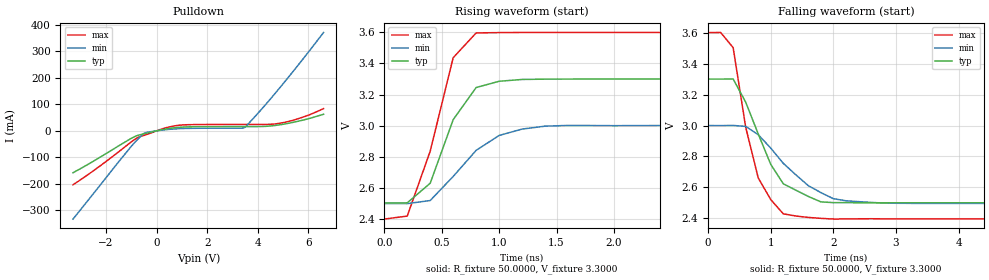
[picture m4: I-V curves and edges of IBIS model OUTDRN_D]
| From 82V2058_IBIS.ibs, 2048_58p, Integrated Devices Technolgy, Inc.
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|   Model OUTDRN_D
[Model]   OUTDRN_D
Model_type   Open_drain
Polarity   Non-Inverting
Vmeas =   1.65V
Vref  =   3.3V
Rref  =   4.7k
C_comp   2.6600pF   2.5500pF   2.7500pF
[Temperature Range]   25.0000   85.0000   -40.0000
[Voltage Range]   3.3000V   3.0000V   3.6000V
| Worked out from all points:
|   slope of the pulldown table from 0 to 0.495 V, typ, clamps not added: 54.8 ohm
|   rising waveform, R_fixture 50.0000, V_fixture 3.3000: 20-80 % time 283ps typ, 419ps min, 268ps max; typ from 2.5 V to 3.3 V
|   falling waveform, R_fixture 50.0000, V_fixture 3.3000: 20-80 % time 531ps typ, 767ps min, 379ps max; typ from 3.3 V to 2.5 V
[Pulldown]
|Voltage   I(typ)   I(min)   I(max)
-3.3V     -158.2mA   -332.9mA   -203.7mA
-2.3V     -103.5mA   -213.8mA   -137.3mA
-1V       -28.38mA   -58.79mA   -41.86mA
-800mV    -19.13mA   -37.45mA   -28.62mA
-500mV    -11.28mA   -9.712mA   -17.25mA
300mV     6.013mA    3.742mA    9.709mA
900mV     13.39mA    8.261mA    21.26mA
3.5V      16.11mA    13.39mA    24.2mA
4.3V      16.95mA    98.13mA    24.36mA
4.9V      23.26mA    166.1mA    29.01mA
5.7V      38.59mA    260.8mA    48.98mA
6.6V      62.62mA    371.4mA    83.82mA
[Ramp]
| variable   typ   min   max
dV/dt_r   0.4794/0.2972n   0.3018/0.3833n   0.7218/0.2409n
dV/dt_f   0.4794/0.5057n   0.3018/0.7074n   0.7218/0.4005n
R_load =   50.0000
[Rising Waveform]
R_fixture=   50.0000
V_fixture=   3.3000
V_fixture_min=  3.0000
V_fixture_max=  3.6000
|time   V(typ)   V(min)   V(max)
0s        2.501V     2.497V     2.397V
200ps     2.502V     2.497V     2.416V
400ps     2.628V     2.517V     2.835V
600ps     3.038V     2.672V     3.437V
800ps     3.245V     2.84V      3.597V
1ns       3.285V     2.936V     3.599V
1.2ns     3.297V     2.977V     3.6V
1.4ns     3.299V     2.996V     3.6V
1.6ns     3.3V       3.001V     3.6V
10ns      3.3V       3V         3.6V
[Falling Waveform]
R_fixture=   50.0000
V_fixture=   3.3000
V_fixture_min=  3.0000
V_fixture_max=  3.6000
|time   V(typ)   V(min)   V(max)
0s        3.3V       3V         3.6V
200ps     3.3V       2.999V     3.601V
400ps     3.3V       3.001V     3.503V
600ps     3.151V     2.994V     2.99V
800ps     2.946V     2.941V     2.662V
1ns       2.749V     2.854V     2.522V
1.2ns     2.624V     2.756V     2.43V
1.6ns     2.542V     2.611V     2.406V
2.2ns     2.502V     2.514V     2.397V
10ns      2.501V     2.497V     2.397V
